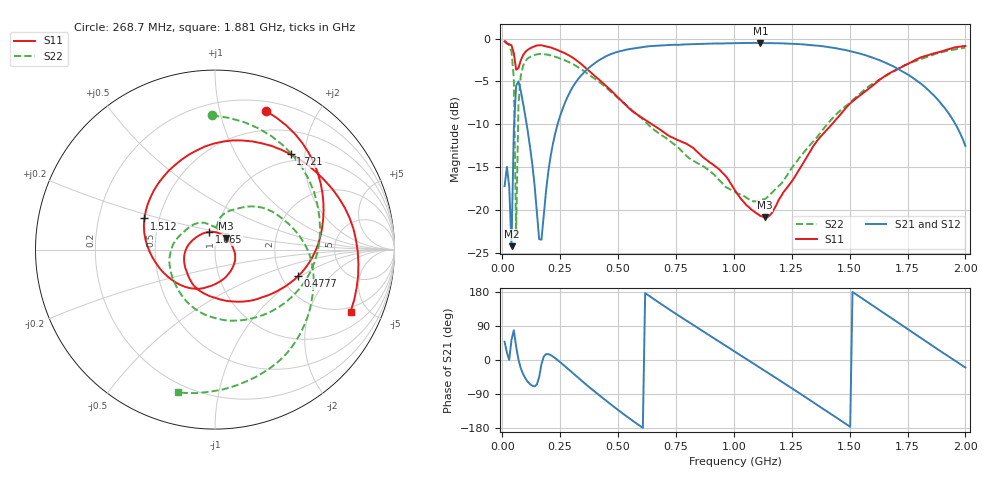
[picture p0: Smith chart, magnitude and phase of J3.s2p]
!Agilent Technologies,E8364B,MY43040703,A.07.50.48
!Agilent E8364B: A.07.50.48
!Date: Friday, November 12, 2021 03:07:44
!Correction: S11(Full 2 Port(1,2))
!S21(Full 2 Port(1,2))
!S12(Full 2 Port(1,2))
!S22(Full 2 Port(1,2))
!S2P File: Measurements: S11, S21, S12, S22:
# Hz S  RI  R 50
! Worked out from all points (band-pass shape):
!   201 points, 10 MHz to 2 GHz, reference 50 ohm
!   highest |S21| = -0.50 dB at 1.114 GHz (marker M1); lowest = -24.3 dB at 39.85 MHz (marker M2)
!   |S21| within 3 dB of the highest: 370.6 MHz to 1.706 GHz (1.335 GHz wide, 129 % of centre)
!   lowest |S11| = -20.9 dB at 1.134 GHz (marker M3), VSWR 1.20, Z = 56.1 + j7.38 ohm
!   |S11| at or under -10 dB: 646.5 MHz to 1.424 GHz (777.4 MHz wide, 75.1 % of centre)
!   |S22| runs from -22.9 to -0.2 dB; largest |S21 - S12| = 0.0023
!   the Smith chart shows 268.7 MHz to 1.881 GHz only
!   S11 on the Smith chart (normalised r, x): 268.7 MHz: 0.29, +1.39; 477.6 MHz: 2.45, -0.96; 1.065 GHz: 0.92, +0.18; 1.512 GHz: 0.41, +0.18; 1.721 GHz: 0.88, +1.73; 1.881 GHz: 1.73, -3.85
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1e7  0.5248 -0.807  0.0915 0.1024  0.0928 0.1016  0.8946 -0.3899
3.985e7  -0.7764 -0.4829  0.0363 0.0494  0.0364 0.0494  -0.1505 -0.8255
4.98e7  -0.8035 -0.1747  0.0587 0.2869  0.0597 0.2871  -0.4828 -0.3331
5.975e7  -0.6538 -0.079  0.43 0.3097  0.4298 0.3097  -0.0147 0.0702
6.97e7  -0.6628 -0.1105  0.5628 0.0156  0.5621 0.0159  0.3261 -0.2421
9.955e7  -0.8227 0.1468  0.2342 -0.2628  0.2336 -0.2622  -0.2281 -0.7033
1.692e8  -0.5119 0.7574  0.0657 -0.0125  0.0658 -0.0126  -0.807 0.1159
2.687e8  0.2839 0.7727  0.4005 -0.1105  0.4009 -0.1103  -0.0156 0.7484
3.483e8  0.5878 0.3731  0.3333 -0.5291  0.3334 -0.5293  0.5218 0.3924
4.7765e8  0.4623 -0.1491  -0.4281 -0.7003  -0.4277 -0.7001  0.3521 -0.3227
6.7665e8  0.076 -0.2871  -0.8 0.4351  -0.7999 0.4349  -0.2423 -0.1388
8.3585e8  -0.1336 -0.1773  0.0378 0.9278  0.0382 0.9289  -0.1424 0.1252
1.005e9  -0.1148 0.0605  0.8744 0.3487  0.8732 0.3485  -0.00286 0.1273
1.0647e9  -0.0313 0.0988  0.9435 -0.0247  0.9428 -0.0252  0.0101 0.1147
1.11445e9  0.0353 0.085  0.8815 -0.3392  0.881 -0.339  0.00274 0.1137
1.13435e9  0.0622 0.0652  0.8247 -0.4539  0.8251 -0.4544  0.00354 0.1155
1.3433e9  -0.0883 -0.2185  -0.3359 -0.8495  -0.3357 -0.8493  0.1114 0.2248
1.51245e9  -0.3929 0.1739  -0.8393 0.00609  -0.8389 0.00675  0.4131 0.1407
1.67165e9  0.1531 0.608  -0.2873 0.6456  -0.2866 0.6444  0.5299 -0.328
1.7214e9  0.4225 0.5306  -0.0401 0.6487  -0.0389 0.6488  0.4514 -0.5087
1.8806e9  0.7552 -0.346  0.3884 0.2082  0.3878 0.2075  -0.207 -0.7959
2e9  0.1455 -0.8948  0.2221 -0.0795  0.2222 -0.0793  -0.7717 -0.4347
